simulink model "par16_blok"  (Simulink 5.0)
settings: Solver=ode45  SolverMode=SingleTasking  StartTime=0.0  StopTime=120.0  MaxStep=0.01  RelTol=1e-3  AbsTol=1e-6

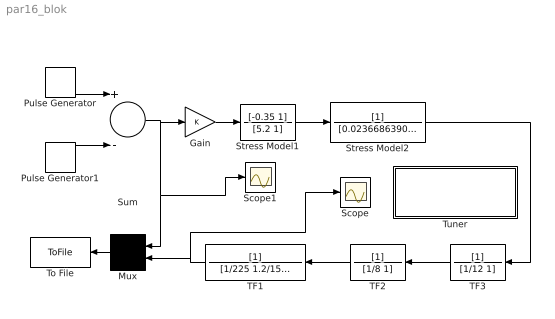
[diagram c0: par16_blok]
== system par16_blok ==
  Gain : Gain
  Mux : Mux  Orientation=left  Inputs=2
  Pulse Generator : DiscretePulseGenerator  PulseType=Time based  Period=40  PulseWidth=50
  Pulse Generator1 : DiscretePulseGenerator  PulseType=Time based  Period=40  PulseWidth=50  PhaseDelay=20
  Scope : Scope
  Scope1 : Scope
  Stress Model1 : TransferFcn  Numerator=[-0.35 1]  Denominator=[5.2 1]
  Stress Model2 : TransferFcn  Denominator=[0.0236686390532544 0.0615384615384615 1]
  Sum : Sum  Inputs=+-
  TF1 : TransferFcn  Orientation=left  Denominator=[1/225 1.2/15 1]
  TF2 : TransferFcn  Orientation=left  Denominator=[1/8 1]
  TF3 : TransferFcn  Orientation=left  Denominator=[1/12 1]
  To File : ToFile  Orientation=left  Filename=bmd16.mat  MatrixName=mbio  SampleTime=0.01
  Tuner : Subsystem  mask(Stress Level 1){name1='par16_blok/Stress Model1', name2='par16_blok/Stress Model2', fname='par16'}
      mask prompts: name1 "'Block Name 1' :"; name2 "'Block Name 2 ' :"; fname "'FileName' :"
      mask init:
      | name1=@1; name2=@2; fname=@3;
      | efname=[fname '.dat'];         eval(['load ' efname]);
      | par=eval(fname);    lp=length(par(1,:));
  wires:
  Gain/1 -> Stress Model1/1
  Stress Model1/1 -> Stress Model2/1
  Stress Model2/1 -> TF3/1
  TF3/1 -> TF2/1
  TF2/1 -> TF1/1
  Mux/1 -> To File/1
  Sum/1 -> Gain/1, Mux/1, Scope1/1
  Pulse Generator1/1 -> Sum/2
  Pulse Generator/1 -> Sum/1
  TF1/1 -> Mux/2, Scope/1

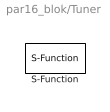
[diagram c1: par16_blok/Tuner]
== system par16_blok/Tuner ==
  S-Function : S-Function  FunctionName=S_bm5_sl  Parameters=name1,name2,par,lp
